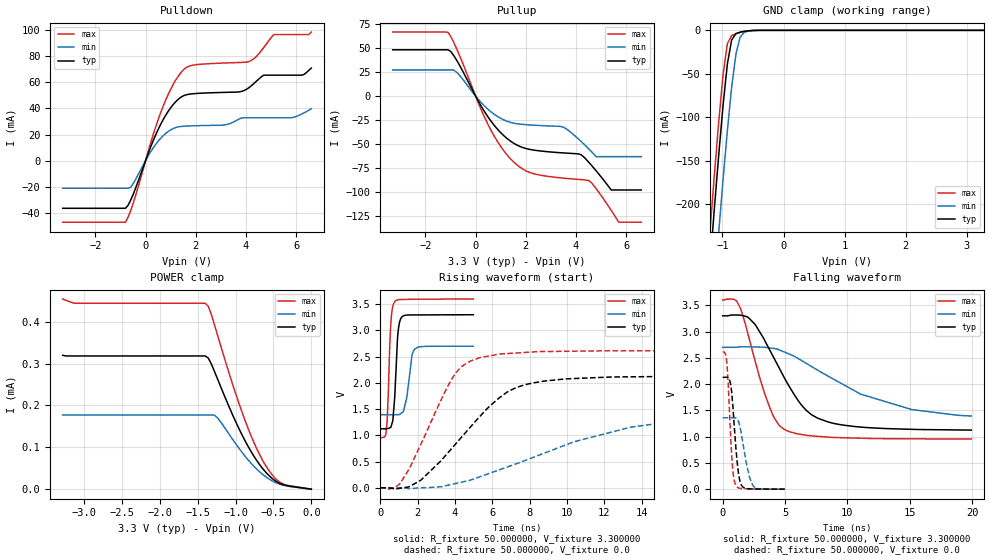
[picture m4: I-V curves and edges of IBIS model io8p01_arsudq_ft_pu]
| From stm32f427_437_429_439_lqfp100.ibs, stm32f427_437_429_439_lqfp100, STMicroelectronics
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|   Model io8p01_arsudq_ft_pu
[Model]  io8p01_arsudq_ft_pu
Model_type I/O
Polarity   Non-Inverting
Enable   Active-Low
Vinl =   0.990000V
Vinh =   2.310000V
Vmeas =  1.650000V
Cref =   50.000000pF
Rref =   100.000000M
Vref =   0.0V
C_comp   2.292100pF   2.228000pF   2.366600pF
[Temperature Range]   25.000000   0.125000k   -40.000000
[Pullup Reference]   3.300000V   2.700000V   3.600000V
[Pulldown Reference]   0.0V   0.0V   0.0V
[POWER Clamp Reference]   3.300000V   2.700000V   3.600000V
[GND Clamp Reference]   0.0V   0.0V   0.0V
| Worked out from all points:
|   slope of the pulldown table from 0 to 0.495 V, typ, clamps not added: 20.9 ohm
|   slope of the pullup table from 0 to 0.495 V, typ, clamps not added: 22.6 ohm
|   GND clamp passes 1 mA (typ) near -0.62 V on its own axis
|   rising waveform, R_fixture 50.000000, V_fixture 3.300000: 20-80 % time 191ps typ, 292ps min, 164ps max; typ from 1.12 V to 3.3 V
|   rising waveform, R_fixture 50.000000, V_fixture 0.0: 20-80 % time 3.35ns typ, 6.85ns min, 2.09ns max; typ from 0.001 V to 2.13 V
|   falling waveform, R_fixture 50.000000, V_fixture 3.300000: 20-80 % time 3.18ns typ, 6.83ns min, 2ns max; typ from 3.3 V to 1.12 V
|   falling waveform, R_fixture 50.000000, V_fixture 0.0: 20-80 % time 434ps typ, 633ps min, 341ps max; typ from 2.13 V to 0.001 V
[Pulldown]
|Voltage   I(typ)   I(min)   I(max)
-3.3V     -36.46mA   -21.09mA   -47.09mA
-800mV    -36.46mA   -21.09mA   -47.09mA
-600mV    -30.5mA    -20.55mA   -38.69mA
700mV     31.4mA     19.11mA    41.71mA
1.2V      45.15mA    25.37mA    61.75mA
1.6V      50.35mA    26.5mA     71.06mA
3.1V      52.28mA    27.26mA    74.76mA
4.1V      55.64mA    32.87mA    75.8mA
4.7V      65.47mA    32.87mA    86.49mA
5.1V      65.47mA    32.87mA    96.56mA
6.2V      65.47mA    35.57mA    96.56mA
6.6V      70.92mA    39.71mA    98.46mA
[Pullup]
|Voltage   I(typ)   I(min)   I(max)
-3.3V     48.4mA     27.38mA    66.91mA
-1.1V     48.4mA     27.38mA    66.69mA
-700mV    35.09mA    23.45mA    46.29mA
500mV     -22.06mA   -14mA      -30.03mA
1.5V      -49.1mA    -28.3mA    -68.56mA
2.2V      -56.04mA   -30.32mA   -80.35mA
3.5V      -59.52mA   -32.65mA   -85.91mA
4.5V      -69.07mA   -55.12mA   -88.37mA
4.8V      -78.21mA   -63.4mA    -96.83mA
5.4V      -98.3mA    -63.4mA    -119.6mA
5.7V      -98.3mA    -63.4mA    -132mA
6.6V      -98.3mA    -63.4mA    -132mA
[GND_clamp]
|Voltage   I(typ)   I(min)   I(max)
-3.3V     -2.318A    -2.397A    -2.291A
-1.2V     -265.5mA   -356.1mA   -227.2mA
-1.13V    -202.6mA   -292.9mA   -164.1mA
-1.06V    -142.2mA   -231.2mA   -104.1mA
-990mV    -85.98mA   -171.6mA   -50.72mA
-920mV    -38.8mA    -115.5mA   -15.28mA
-850mV    -11.08mA   -65.6mA    -6.001mA
-780mV    -3.782mA   -27.42mA   -3.876mA
-710mV    -2.086mA   -7.69mA    -2.381mA
-640mV    -1.147mA   -2.118mA   -1.22mA
-570mV    -523.9uA   -798.4uA   -476.8uA
3.28V     0A         0A         0A
[POWER_clamp]
|Voltage   I(typ)   I(min)   I(max)
-3.28V    319.9uA    177.1uA    454.3uA
-3.12V    318.3uA    177.1uA    444.3uA
-1.4V     318.3uA    177.1uA    444.3uA
-1.36V    313.4uA    177.1uA    437.2uA
-1.28V    282.3uA    177.1uA    394.1uA
-1.24V    264.6uA    170.9uA    369.7uA
-920mV    131.9uA    89.35uA    187.2uA
-760mV    79.47uA    55.13uA    112.7uA
-640mV    48.78uA    35.04uA    68.06uA
-520mV    26.21uA    20.11uA    35uA
-400mV    12.52uA    10.81uA    14.88uA
0V        0A         0A         0A
[Ramp]
| variable   typ   min   max
dV/dt_r  1.27759/3.34592n   0.79935/6.85212n   1.56694/2.09211n
dV/dt_f  1.30158/3.17847n   0.73980/6.80055n   1.58711/1.99753n
R_load = 50.000000
[Rising Waveform]
R_fixture= 50.000000
V_fixture= 3.300000
V_fixture_min= 2.700000
V_fixture_max= 3.600000
|time   V(typ)   V(min)   V(max)
0s        1.125V     1.393V     955.6mV
300.3ps   1.127V     1.393V     1.017V
370.4ps   1.129V     1.393V     1.282V
500.5ps   1.143V     1.393V     2.643V
590.6ps   1.183V     1.393V     3.256V
760.8ps   1.669V     1.392V     3.541V
940.9ps   2.924V     1.395V     3.584V
1.161ns   3.259V     1.432V     3.591V
1.842ns   3.296V     2.645V     3.595V
4.985ns   3.3V       2.7V       3.599V
[Rising Waveform]
R_fixture= 50.000000
V_fixture= 0.0
V_fixture_min= 0.0
V_fixture_max= 0.0
|time   V(typ)   V(min)   V(max)
0s        1.446mV    1.248mV    1.82mV
1.081ns   -5.878mV   -926.7uV   94.72mV
2.162ns   142.7mV    818.2uV    820.1mV
3.724ns   708.7mV    57.78mV    2.008V
4.244ns   921.1mV    98.97mV    2.27V
4.845ns   1.165V     148.7mV    2.418V
6.767ns   1.819V     393mV      2.56V
8.168ns   1.999V     577.4mV    2.591V
13.41ns   2.116V     1.156V     2.612V
19.94ns   2.129V     1.36V      2.612V
[Falling Waveform]
R_fixture= 50.000000
V_fixture= 3.300000
V_fixture_min= 2.700000
V_fixture_max= 3.600000
|time   V(typ)   V(min)   V(max)
0s        3.3V       2.7V       3.599V
880.9ps   3.315V     2.7V       3.615V
1.441ns   3.311V     2.71V      3.433V
2.603ns   3.136V     2.707V     2.439V
3.724ns   2.67V      2.691V     1.586V
4.965ns   2.11V      2.609V     1.136V
6.727ns   1.496V     2.391V     1.026V
8.408ns   1.284V     2.158V     992mV
15.18ns   1.14V      1.516V     959.4mV
19.94ns   1.125V     1.393V     955.6mV
[Falling Waveform]
R_fixture= 50.000000
V_fixture= 0.0
V_fixture_min= 0.0
V_fixture_max= 0.0
|time   V(typ)   V(min)   V(max)
0s        2.129V     1.36V      2.612V
300.3ps   2.131V     1.359V     2.474V
450.5ps   2.12V      1.359V     1.951V
620.6ps   2.016V     1.359V     1.082V
830.8ps   1.523V     1.361V     321.6mV
1.041ns   830.8mV    1.354V     82.59mV
1.451ns   103mV      1.118V     14.65mV
1.872ns   14.37mV    524mV      7.563mV
2.422ns   5.641mV    73.54mV    4.639mV
4.985ns   1.446mV    1.248mV    1.82mV
